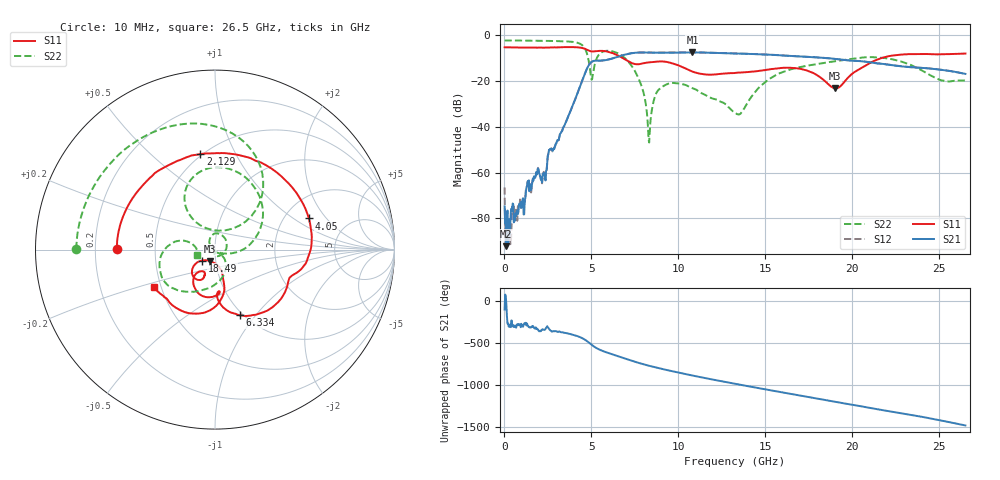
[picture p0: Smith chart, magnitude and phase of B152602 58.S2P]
!  2-Port S-parameters saved by WinCal
! VAR MeasName=S-Parameters (CALIBRATED_DATA) read from VNA (N5242A)
! VAR MeasDate=2016-1-5 16:34:11
! VAR NAME=B152602 58
! VAR FILENAME=B152602 58.S2P
! VAR DATE=2016-1-5 16:34:11
! VAR PHYS_PORTS=1,2
# Hz S DB R 50
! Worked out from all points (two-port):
!   801 points, 10 MHz to 26.5 GHz, reference 50 ohm
!   highest |S21| = -7.46 dB at 10.8 GHz (marker M1); lowest = -92.2 dB at 109.3 MHz (marker M2)
!   |S21| within 3 dB of the highest: 6.04 GHz to 19.2 GHz (13.16 GHz wide, 104 % of centre)
!   lowest |S11| = -23.2 dB at 19.02 GHz (marker M3), VSWR 1.15, Z = 47.1 - j6.11 ohm
!   |S11| at or under -10 dB: 6.812 GHz to 21.66 GHz (14.85 GHz wide, 104 % of centre)
!   |S22| runs from -46.9 to -2.2 dB; largest |S21 - S12| = 0.0031
!   S11 on the Smith chart (normalised r, x): 10 MHz: 0.29, +0.00; 2.129 GHz: 0.49, +0.73; 4.05 GHz: 2.70, +1.35; 6.334 GHz: 0.97, -0.84; 18.49 GHz: 0.86, -0.11; 26.5 GHz: 0.46, -0.23
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1e7  -5.25 179.6  -74.81 -104.1  -66.53 30.7  -2.24 179.8
1.093375e8  -5.24 175.8  -92.21 -38.8  -87.22 82.5  -2.24 178.3
6.7225e8  -5.30 154.3  -78.99 40.2  -77.05 53.1  -2.27 169.6
1.367612e9  -5.31 128.2  -64.91 59.7  -64.52 66.1  -2.33 158.7
2.1292e9  -5.37 98.6  -62.84 14.6  -62.33 16.9  -2.41 146.0
4.049725e9  -5.18 18.3  -28.30 -49.7  -28.29 -49.5  -3.01 97.2
4.447075e9  -5.50 -0.8  -20.26 -81.6  -20.25 -81.5  -4.15 74.7
5.0431e9  -7.06 -20.9  -11.48 -168.3  -11.47 -168.2  -19.07 99.0
5.506675e9  -6.77 -35.4  -11.06 135.5  -11.07 135.7  -7.87 110.6
6.334488e9  -8.13 -69.0  -9.81 74.0  -9.79 74.1  -7.27 65.6
7.625875e9  -12.65 -84.7  -7.58 -13.0  -7.55 -13.0  -17.51 -4.3
7.990112e9  -12.22 -84.3  -7.53 -35.2  -7.52 -35.1  -24.85 -22.4
8.321238e9  -11.82 -88.7  -7.58 -53.3  -7.55 -53.4  -46.88 -150.1
8.851038e9  -11.44 -98.3  -7.60 -80.3  -7.56 -80.4  -23.91 118.0
1.080468e10  -15.84 -127.3  -7.46 -168.6  -7.45 -168.7  -23.08 22.0
1.3255e10  -16.45 -112.0  -7.92 92.6  -7.90 92.5  -33.93 -89.5
1.544042e10  -14.66 -114.6  -8.57 10.1  -8.53 10.0  -18.10 -61.4
1.769208e10  -16.24 -141.8  -9.52 -72.7  -9.51 -72.5  -12.93 -103.2
1.848678e10  -20.49 -139.6  -9.96 -102.1  -9.93 -102.2  -11.94 -113.3
1.901658e10  -23.16 -111.8  -10.33 -121.9  -10.30 -121.9  -11.36 -119.8
2.209604e10  -9.11 -97.8  -12.90 126.5  -12.81 126.3  -10.19 -170.9
2.65e10  -7.97 -148.3  -16.86 -43.3  -16.86 -43.5  -19.79 -164.1
